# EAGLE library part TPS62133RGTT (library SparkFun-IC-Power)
3-17V, 2A Step Down Converter(IC-11155)
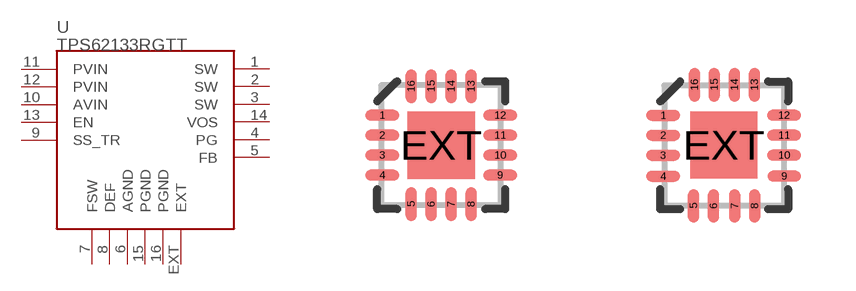
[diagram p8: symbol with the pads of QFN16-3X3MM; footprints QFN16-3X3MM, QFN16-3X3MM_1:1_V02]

Designator prefix U

## TPS62133RGTTV01  [QFN16-3X3MM]
1  SW
2  SW
3  SW
4  PG
5  FB
6  AGND
7  FSW
8  DEF
9  SS_TR
10  AVIN
11  PVIN
12  PVIN
13  EN
14  VOS
15  PGND
16  PGND
EXT  EXT

## TPS62133RGTTV02  [QFN16-3X3MM_1:1_V02]
Pads as for QFN16-3X3MM

## TPS62133RGTT"" (PROD_ID: IC-11155)  [QFN16-3X3MM_1:1_V03]
Pads as for QFN16-3X3MM

## Footprint QFN16-3X3MM (pad centres in mm)
3mm x 3mm QFN 16 pin
smd 0.85 x 0.28: 1 -1.475,0.75; 2 -1.475,0.25; 3 -1.475,-0.25; 4 -1.475,-0.75; 9 1.475,-0.75; 10 1.475,-0.25; 11 1.475,0.25; 12 1.475,0.75
smd 0.28 x 0.85: 5 -0.75,-1.475; 6 -0.25,-1.475; 7 0.25,-1.475; 8 0.75,-1.475; 13 0.75,1.475; 14 0.25,1.475; 15 -0.25,1.475; 16 -0.75,1.475
smd 1.68 x 1.68: EXT 0,0

## Footprint QFN16-3X3MM_1:1_V02 (pad centres in mm)
smd 0.85 x 0.28: 1 -1.524,0.75; 2 -1.524,0.253; 3 -1.529,-0.25; 4 -1.527,-0.774; 9 1.503,-0.77; 10 1.498,-0.245; 11 1.498,0.255; 12 1.495,0.755
smd 0.28 x 0.85: 5 -0.765,-1.513; 6 -0.265,-1.513; 7 0.263,-1.513; 8 0.763,-1.513; 13 0.758,1.518; 14 0.258,1.518; 15 -0.247,1.518; 16 -0.742,1.518
smd 1.68 x 1.68: EXT -0.009,0.008

## Footprint QFN16-3X3MM_1:1_V03 (pad centres in mm)
smd 0.85 x 0.28: 1 -1.524,0.75; 2 -1.524,0.253; 3 -1.529,-0.25; 4 -1.527,-0.774; 9 1.503,-0.77; 10 1.498,-0.245; 11 1.498,0.255; 12 1.495,0.755
smd 0.28 x 0.85: 5 -0.765,-1.513; 6 -0.265,-1.513; 7 0.263,-1.513; 8 0.763,-1.513; 13 0.758,1.518; 14 0.258,1.518; 15 -0.247,1.518; 16 -0.742,1.518
smd 1.68 x 1.68: EXT -0.009,0.008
